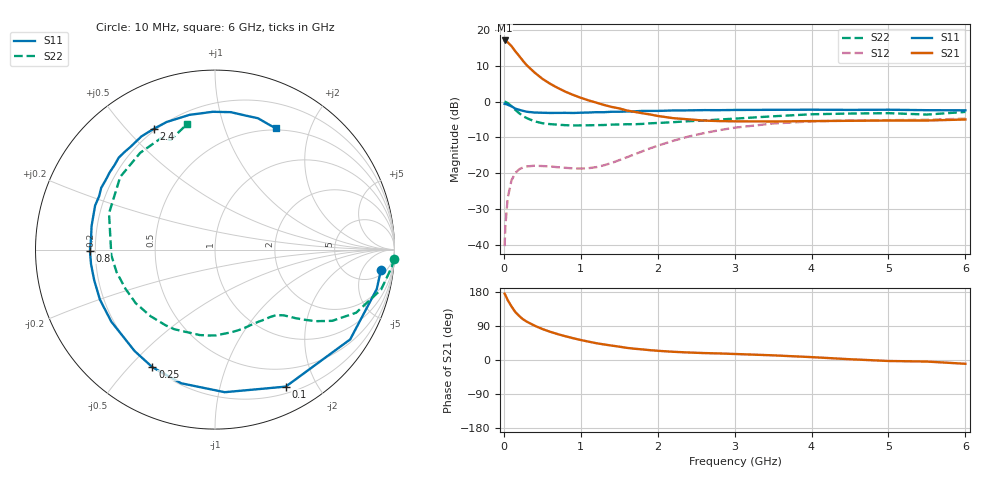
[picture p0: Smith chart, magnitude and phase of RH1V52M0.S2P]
! SIEMENS Small Signal Semiconductors
! BFR106
! Si NPN RF Bipolar Junction Transistor in SOT23
! VCE = 1.5 V  IC = 2 mA
! Common Emitter S-Parameters:  August  1996
# GHz  S  MA  R  50
!  f  S11  S21  S12  S22
! GHz  MAG  ANG  MAG  ANG  MAG  ANG  MAG  ANG
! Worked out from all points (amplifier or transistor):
!   36 points, 10 MHz to 6 GHz, reference 50 ohm
!   highest |S21| = 17.0 dB at 10 MHz (marker M1)
!   |S21| within 3 dB of that: start of sweep to 148.9 MHz
!   unconditionally stable (mu >= 1): 773.7 MHz to end of sweep
!   at 250 MHz: K = 0.33, MSG = 14.8 dB, |S12| = -18.3 dB
!   at 1.4 GHz: K = 1.32, MAG = 4.4 dB, |S12| = -17.1 dB
!   at 6 GHz: K = 1.02, MAG = -1.1 dB, |S12| = -4.8 dB
!   S11 on the Smith chart (normalised r, x): 10 MHz: 7, -12; 100 MHz: 0.28, -1.61; 250 MHz: 0.20, -0.58; 800 MHz: 0.18, -0.00; 2.4 GHz: 0.19, +0.60; 6 GHz: 0.48, +1.52
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0.01  0.9315 -7.0  7.096 174.9  0.0097 86.4  0.9977 -2.9
0.02  0.9277 -13.7  7.044 171.4  0.0186 83.9  0.9897 -5.6
0.05  0.9042 -33.6  6.687 158.2  0.0454 71.5  0.9521 -13.5
0.1  0.8591 -62.7  5.908 141.2  0.0803 56.8  0.8613 -24.1
0.15  0.7963 -86.1  5.006 126.3  0.1016 44.9  0.7641 -31.3
0.2  0.7682 -104.2  4.304 116.1  0.1141 37.5  0.6885 -35.4
0.25  0.7423 -118.0  3.68 107.3  0.1211 31.4  0.6261 -38.5
0.3  0.7211 -128.4  3.189 101.0  0.1252 28.1  0.5873 -40.5
0.4  0.7035 -145.2  2.537 90.5  0.1278 23.2  0.5303 -43.7
0.5  0.6991 -156.5  2.079 81.9  0.1266 20.8  0.4997 -46.9
0.6  0.6944 -165.7  1.775 74.6  0.1252 20.2  0.4856 -50.6
0.8  0.6969 -179.5  1.373 62.7  0.1196 23.4  0.4691 -59.0
1.1  0.7039 164.2  1.04 48.5  0.1182 36.1  0.4676 -73.6
1.6  0.7278 143.6  0.751 32.0  0.1678 56.2  0.4838 -100.3
2.2  0.7522 123.0  0.588 21.7  0.2843 56.4  0.5163 -134.1
2.4  0.7545 116.8  0.566 19.8  0.3258 53.3  0.5331 -145.9
3  0.7641 100.7  0.531 15.9  0.4329 40.4  0.5785 -176.9
3.5  0.7679 90.9  0.528 12.3  0.4951 29.3  0.6241 161.1
4.5  0.7659 77.1  0.54 2.0  0.5443 10.2  0.6814 127.7
5  0.7701 71.9  0.545 -2.6  0.5513 3.0  0.6899 115.8
5.5  0.7587 66.7  0.545 -4.1  0.5576 -0.2  0.6593 111.9
6  0.7559 63.2  0.563 -10.0  0.5786 -7.5  0.7178 102.4
